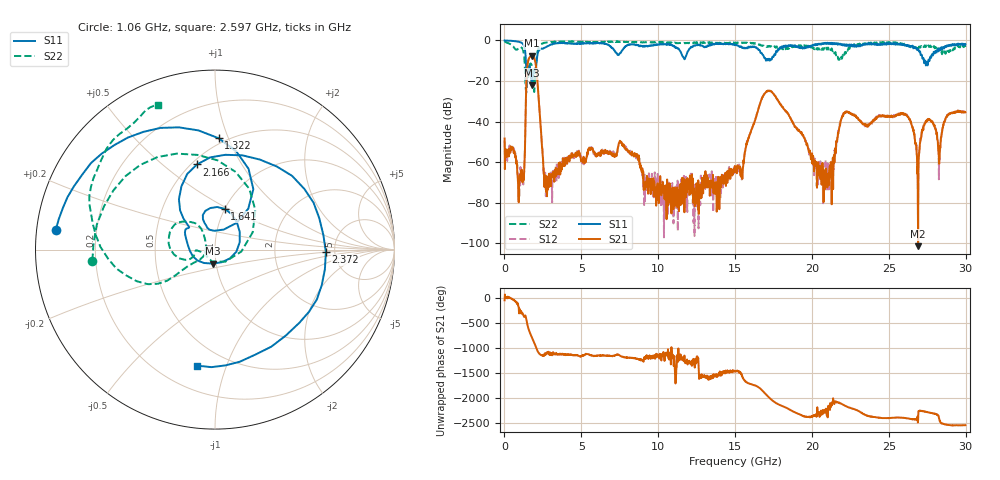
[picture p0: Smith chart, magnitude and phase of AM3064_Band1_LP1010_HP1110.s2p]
# Hz S DB R 50.0
!freq dBS11 angS11 dBS21 angS21 dBS12 angS12 dBS22 angS22
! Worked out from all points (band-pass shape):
!   1600 points, 10 MHz to 29.98 GHz, reference 50 ohm
!   highest |S21| = -7.60 dB at 1.791 GHz (marker M1); lowest = -101.4 dB at 26.91 GHz (marker M2)
!   |S21| within 3 dB of the highest: 1.526 GHz to 2.005 GHz (479 MHz wide, 27.1 % of centre)
!   lowest |S11| = -22.1 dB at 1.791 GHz (marker M3), VSWR 1.17, Z = 48.1 - j7.5 ohm
!   |S11| at or under -10 dB: 1.393 GHz to 2.099 GHz (706.7 MHz wide, 40.5 % of centre); 27.2822 GHz to 27.35143 GHz (69.24 MHz wide, 0.253 % of centre); 27.36 GHz to 27.57 GHz (207.9 MHz wide, 0.757 % of centre)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
!   |S22| runs from -25.8 to -0.4 dB; largest |S21 - S12| = 0.0071
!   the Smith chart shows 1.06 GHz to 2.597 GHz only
!   S11 on the Smith chart (normalised r, x): 1.06 GHz: 0.06, +0.06; 1.322 GHz: 0.46, +0.92; 1.641 GHz: 1.00, +0.48; 2.166 GHz: 0.53, +0.66; 2.372 GHz: 4.22, -0.19; 2.597 GHz: 0.35, -0.80
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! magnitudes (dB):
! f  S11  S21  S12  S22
! 10 MHz  0.0  -48.4  -49.5  -0.4
! 1.06 GHz  -1.0  -65.1  -67.4  -3.3
! 1.322 GHz  -4.1  -57.3  -55.9  -12.7
! 1.641 GHz  -12.6  -8.3  -8.3  -12.1
! 1.791 GHz  -22.1  -7.6  -7.6  -13.0
! 2.166 GHz  -6.3  -22.3  -22.3  -5.0
! 2.372 GHz  -4.2  -44.3  -43.4  -1.9
! 2.597 GHz  -3.7  -72.3  -64.3  -1.2
! 5.015 GHz  -1.4  -59.6  -59.1  -0.8
! 7.601 GHz  -5.6  -50.1  -50.2  -0.7
! 10 GHz  -2.0  -71.7  -69.0  -1.0
! 15 GHz  -2.1  -64.9  -64.2  -1.4
! 17.16 GHz  -9.5  -24.9  -24.8  -3.2
! 19.99 GHz  -2.9  -57.4  -57.7  -3.2
! 20.91 GHz  -1.4  -63.3  -74.0  -3.7
! 22.13 GHz  -2.4  -35.9  -35.6  -6.2
! 25 GHz  -1.3  -37.3  -37.4  -1.1
! 26.25 GHz  -2.9  -37.8  -37.8  -2.4
! 26.91 GHz  -4.2  -101.4  -77.6  -3.8
! 27.49 GHz  -10.8  -39.7  -39.7  -3.0
! 28.28 GHz  -4.1  -60.9  -58.1  -4.2
! 29.98 GHz  -1.8  -35.4  -35.2  -3.2
